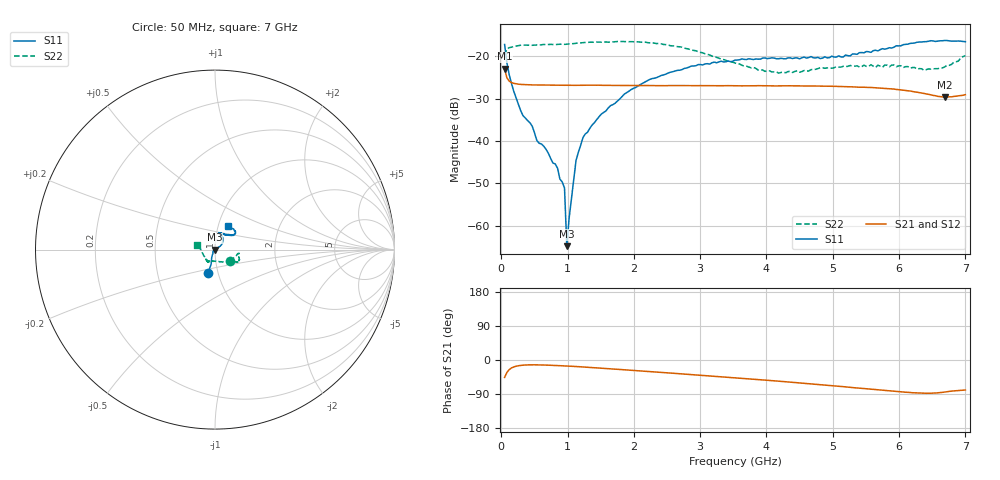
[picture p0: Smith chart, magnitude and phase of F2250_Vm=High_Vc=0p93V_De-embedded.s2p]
! Integrated Device Technology
! Corporate Headquarters
! 6024 Silver Creek Valley Road
! San Jose, CA 95138  USA
! Phone:  1-408-284-8200
! Toll Free:  1-800-223-1366
! Webpage:  http://www.idt.com/
! Timing and RF Division
! 515 Groton Road, Suite 102
! Westford, MA 01886-6024
! Device:  F2250
! Description: Voltage Variable RF Attenuator
! Frequency:  50.0 -  6000.00 MHz
! Package:  3x3 mm Thin QFN Plastic Package: 16 pin
! Ports:  2 RF, 3 DC
!  Pin  1  = GND
!  Pin  2  = NC
!  Pin  3  = RF1  = Port 1
!  Pin  4  = NC
!  Pin  5  = GND
!  Pin  6  = GND
!  Pin  7  = GND
!  Pin  8  = GND
!  Pin  9  = NC
!  Pin 10  = RF2  = Port 2
!  Pin 11  = NC
!  Pin 12  = GND
!  Pin 13  = GND
!  Pin 14  = VCNTRL
!  Pin 15  = VDD
!  Pin 16  = VMODE
! Vcntrl:  0.930 Volts
! Vmode:  +3.300 Volts
! Vdd:  +3.30  Volts
! Current:  1.317 mA
! Data:  The device was measured on a the F2250 evaluation board which has
!  individual transmission lines to the RF pins.  Data was collected
!  using a calibrated network analyzer.  The evaluation board was
!  de-embedded using a TRL calibration technique.
!  The reference plane is the edge of the package pin.
! Misc:  SN 10
!  Action Tracker AT0258
! Date Measured:  2014-11-26
! Date:  2015-10-15  MJV
! Note:
!  Integrated Device Technology supplies this data as a sample of measured
!  data at the package pin for this product.  Your particular data for this
!  product may vary.
!  Data was taken at 25 degrees C.
!  Integrated Device Technology reserves the right to change this data at anytime.
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# GHz S dB R 50
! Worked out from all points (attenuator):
!   201 points, 50 MHz to 7 GHz, reference 50 ohm
!   highest |S21| = -22.91 dB at 50 MHz (marker M1); lowest = -29.6 dB at 6.687 GHz (marker M2)
!   lowest |S11| = -64.8 dB at 988.2 MHz (marker M3), VSWR 1.00, Z = 49.9 - j0.0171 ohm
!   |S11| at or under -10 dB: start of sweep to end of sweep
!   |S22| runs from -23.9 to -16.5 dB; largest |S21 - S12| = 0.00017
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0.05  -17.19 -106.7  -22.91 -45.8  -22.90 -45.8  -19.80 -37.6
0.1195  -24.32 -108.6  -25.82 -25.4  -25.83 -25.4  -17.92 -12.1
0.29325  -32.85 -119.6  -26.61 -14.2  -26.61 -14.2  -17.35 -9.4
0.467  -36.50 -136.8  -26.73 -12.7  -26.71 -12.7  -17.36 -9.7
0.5365  -39.87 -142.9  -26.73 -12.8  -26.74 -12.8  -17.29 -11.0
0.8145  -45.40 173.7  -26.81 -14.4  -26.81 -14.4  -17.20 -15.3
0.9535  -51.07 -177.4  -26.81 -15.5  -26.80 -15.5  -17.15 -17.6
0.98825  -64.83 -162.7  -26.82 -15.9  -26.82 -15.9  -17.11 -18.1
1.023  -58.23 31.7  -26.81 -16.2  -26.81 -16.2  -17.03 -18.3
1.12725  -44.58 25.8  -26.82 -17.2  -26.81 -17.2  -16.89 -19.7
1.2315  -39.18 24.3  -26.81 -18.3  -26.80 -18.3  -16.73 -21.5
1.5095  -33.61 31.7  -26.83 -21.7  -26.82 -21.7  -16.64 -23.7
1.857  -28.88 34.1  -26.83 -25.9  -26.83 -25.9  -16.47 -26.5
2.37825  -24.73 43.3  -26.89 -32.3  -26.90 -32.3  -16.93 -29.7
2.86475  -22.28 54.9  -26.92 -38.4  -26.94 -38.4  -18.49 -34.4
3.525  -20.87 70.1  -26.92 -47.0  -26.94 -47.1  -21.56 -55.5
4.18525  -20.53 76.4  -26.95 -55.8  -26.94 -55.9  -23.94 -89.4
4.7065  -20.32 71.1  -26.98 -63.6  -26.98 -63.6  -23.08 -111.0
5.85325  -17.94 39.7  -27.64 -81.4  -27.62 -81.5  -22.45 -124.1
6.3745  -16.52 40.3  -28.71 -87.7  -28.72 -87.8  -23.29 -141.6
6.68725  -16.24 47.2  -29.61 -84.6  -29.60 -84.7  -22.49 -174.1
7  -16.51 61.9  -29.04 -79.3  -29.07 -79.3  -19.81 165.9
